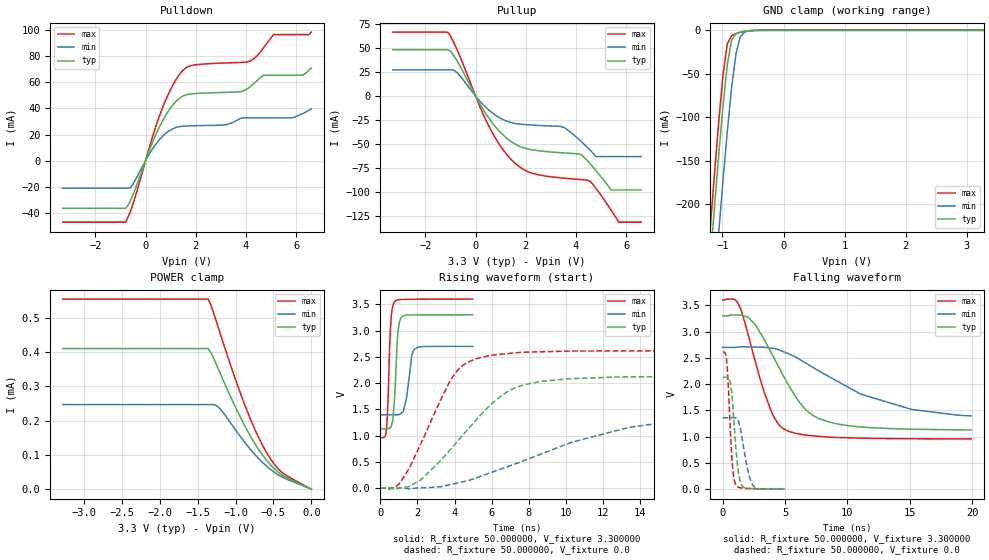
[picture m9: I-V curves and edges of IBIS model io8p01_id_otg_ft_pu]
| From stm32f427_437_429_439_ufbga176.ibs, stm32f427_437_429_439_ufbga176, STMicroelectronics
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|   Model io8p01_id_otg_ft_pu
[Model]  io8p01_id_otg_ft_pu
Model_type I/O
Polarity   Non-Inverting
Enable   Active-Low
Vinl =   0.990000V
Vinh =   2.310000V
Vmeas =  1.650000V
Cref =   50.000000pF
Rref =   100.000000M
Vref =   0.0V
C_comp   2.283100pF   2.214500pF   2.357400pF
[Temperature Range]   25.000000   0.125000k   -40.000000
[Pullup Reference]   3.300000V   2.700000V   3.600000V
[Pulldown Reference]   0.0V   0.0V   0.0V
[POWER Clamp Reference]   3.300000V   2.700000V   3.600000V
[GND Clamp Reference]   0.0V   0.0V   0.0V
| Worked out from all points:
|   slope of the pulldown table from 0 to 0.495 V, typ, clamps not added: 20.9 ohm
|   slope of the pullup table from 0 to 0.495 V, typ, clamps not added: 22.6 ohm
|   GND clamp passes 1 mA (typ) near -0.62 V on its own axis
|   rising waveform, R_fixture 50.000000, V_fixture 3.300000: 20-80 % time 191ps typ, 292ps min, 163ps max; typ from 1.13 V to 3.3 V
|   rising waveform, R_fixture 50.000000, V_fixture 0.0: 20-80 % time 3.36ns typ, 6.88ns min, 2.1ns max; typ from 0.005 V to 2.13 V
|   falling waveform, R_fixture 50.000000, V_fixture 3.300000: 20-80 % time 3.18ns typ, 6.84ns min, 2ns max; typ from 3.3 V to 1.13 V
|   falling waveform, R_fixture 50.000000, V_fixture 0.0: 20-80 % time 436ps typ, 633ps min, 343ps max; typ from 2.13 V to 0.005 V
[Pulldown]
|Voltage   I(typ)   I(min)   I(max)
-3.3V     -36.46mA   -21.09mA   -47.09mA
-800mV    -36.46mA   -21.09mA   -47.09mA
-600mV    -30.5mA    -20.54mA   -38.69mA
700mV     31.4mA     19.11mA    41.71mA
1.2V      45.15mA    25.37mA    61.75mA
1.6V      50.35mA    26.5mA     71.05mA
3.1V      52.28mA    27.26mA    74.75mA
4.1V      55.64mA    32.83mA    75.8mA
4.7V      65.4mA     32.83mA    86.49mA
5.1V      65.4mA     32.83mA    96.56mA
6.2V      65.4mA     35.57mA    96.56mA
6.6V      70.92mA    39.71mA    98.46mA
[Pullup]
|Voltage   I(typ)   I(min)   I(max)
-3.3V     48.4mA     27.38mA    66.92mA
-1.1V     48.4mA     27.38mA    66.69mA
-700mV    35.09mA    23.45mA    46.28mA
500mV     -22.06mA   -13.99mA   -30.02mA
1.5V      -49.09mA   -28.3mA    -68.55mA
2.2V      -56.03mA   -30.32mA   -80.33mA
3.5V      -59.51mA   -32.64mA   -85.89mA
4.5V      -69.05mA   -55.11mA   -88.35mA
4.8V      -78.2mA    -63.4mA    -96.8mA
5.4V      -98.3mA    -63.4mA    -119.5mA
5.7V      -98.3mA    -63.4mA    -132mA
6.6V      -98.3mA    -63.4mA    -132mA
[GND_clamp]
|Voltage   I(typ)   I(min)   I(max)
-3.3V     -2.318A    -2.397A    -2.291A
-1.2V     -265.5mA   -356.1mA   -227.2mA
-1.13V    -202.7mA   -292.9mA   -164.1mA
-1.06V    -142.2mA   -231.2mA   -104.1mA
-990mV    -85.98mA   -171.6mA   -50.73mA
-920mV    -38.81mA   -115.5mA   -15.3mA
-850mV    -11.1mA    -65.61mA   -6.021mA
-780mV    -3.796mA   -27.43mA   -3.892mA
-710mV    -2.096mA   -7.699mA   -2.393mA
-640mV    -1.154mA   -2.125mA   -1.227mA
-570mV    -528.1uA   -803.6uA   -480.7uA
3.28V     0A         0A         0A
[POWER_clamp]
|Voltage   I(typ)   I(min)   I(max)
-3.28V    410.1uA    246.5uA    554.5uA
-1.36V    410.1uA    246.5uA    554.5uA
-1.32V    396.3uA    246.5uA    534.1uA
-1.28V    377.3uA    246.5uA    507.5uA
-1.2V     337.1uA    233.5uA    452.5uA
-1.04V    257.7uA    185.3uA    345.3uA
-880mV    185.4uA    137uA      247uA
-760mV    138.3uA    104.8uA    181.8uA
-640mV    98.44uA    77.14uA    126.4uA
-520mV    66.65uA    54.47uA    82.45uA
-400mV    43.68uA    37.32uA    51.43uA
0V        0A         0A         0A
[Ramp]
| variable   typ   min   max
dV/dt_r  1.27644/3.36175n   0.79944/6.89481n   1.56531/2.09868n
dV/dt_f  1.29912/3.18017n   0.73752/6.80411n   1.58470/2.00306n
R_load = 50.000000
[Rising Waveform]
R_fixture= 50.000000
V_fixture= 3.300000
V_fixture_min= 2.700000
V_fixture_max= 3.600000
|time   V(typ)   V(min)   V(max)
0s        1.129V     1.397V     959.6mV
300.3ps   1.131V     1.397V     1.021V
370.4ps   1.133V     1.397V     1.286V
500.5ps   1.147V     1.397V     2.65V
590.6ps   1.187V     1.397V     3.261V
760.8ps   1.674V     1.396V     3.542V
940.9ps   2.928V     1.399V     3.585V
1.161ns   3.26V      1.436V     3.591V
1.842ns   3.296V     2.646V     3.595V
4.985ns   3.3V       2.7V       3.599V
[Rising Waveform]
R_fixture= 50.000000
V_fixture= 0.0
V_fixture_min= 0.0
V_fixture_max= 0.0
|time   V(typ)   V(min)   V(max)
0s        4.851mV    4.397mV    5.425mV
480.5ps   2.343mV    4.324mV    -16.12mV
1.081ns   5.672mV    2.288mV    109.6mV
2.162ns   154.3mV    9.636mV    831.5mV
3.884ns   782.7mV    78.99mV    2.108V
5.085ns   1.269V     187.3mV    2.455V
6.887ns   1.845V     415.5mV    2.562V
8.769ns   2.036V     665.8mV    2.597V
13.45ns   2.119V     1.162V     2.613V
19.94ns   2.131V     1.363V     2.614V
[Falling Waveform]
R_fixture= 50.000000
V_fixture= 3.300000
V_fixture_min= 2.700000
V_fixture_max= 3.600000
|time   V(typ)   V(min)   V(max)
0s        3.3V       2.7V       3.599V
880.9ps   3.315V     2.7V       3.615V
1.441ns   3.311V     2.71V      3.433V
2.603ns   3.136V     2.707V     2.442V
3.724ns   2.672V     2.691V     1.593V
4.965ns   2.114V     2.609V     1.141V
6.807ns   1.484V     2.381V     1.027V
8.529ns   1.283V     2.144V     994mV
15.14ns   1.144V     1.522V     963.5mV
19.94ns   1.129V     1.397V     959.6mV
[Falling Waveform]
R_fixture= 50.000000
V_fixture= 0.0
V_fixture_min= 0.0
V_fixture_max= 0.0
|time   V(typ)   V(min)   V(max)
0s        2.131V     1.363V     2.614V
300.3ps   2.132V     1.363V     2.475V
620.6ps   2.018V     1.362V     1.091V
830.8ps   1.526V     1.364V     334mV
1.031ns   868.7mV    1.357V     102.1mV
1.261ns   322.5mV    1.295V     40.97mV
1.451ns   112.8mV    1.121V     30.01mV
2.132ns   18.85mV    248.5mV    15.59mV
2.432ns   15.89mV    74.09mV    12.61mV
4.985ns   4.851mV    4.397mV    5.425mV
